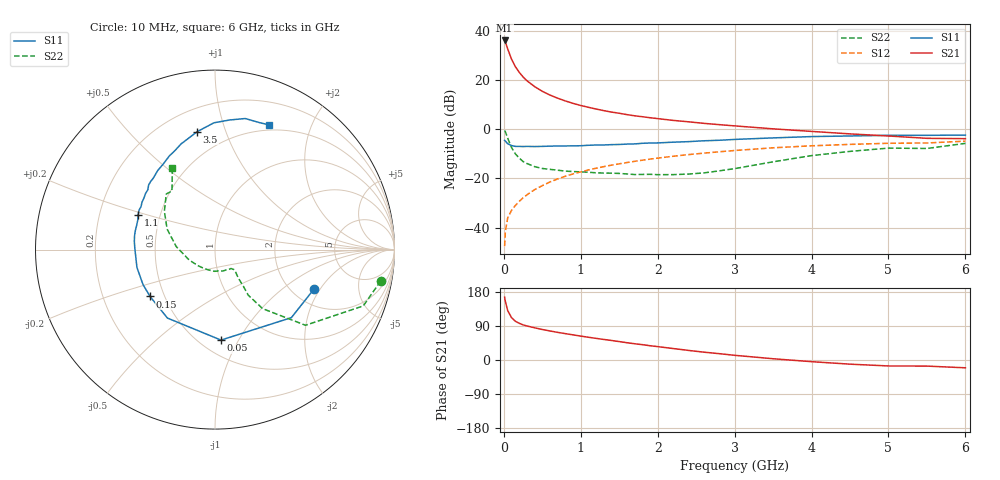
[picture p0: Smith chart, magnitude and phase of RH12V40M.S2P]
! SIEMENS Small Signal Semiconductors
! BFR106
! Si NPN RF Bipolar Junction Transistor in SOT23
! VCE = 12 V  IC = 40 mA
! Common Emitter S-Parameters:  August  1996
# GHz  S  MA  R  50
!  f  S11  S21  S12  S22
! GHz  MAG  ANG  MAG  ANG  MAG  ANG  MAG  ANG
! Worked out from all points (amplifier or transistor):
!   36 points, 10 MHz to 6 GHz, reference 50 ohm
!   highest |S21| = 36.0 dB at 10 MHz (marker M1)
!   |S21| within 3 dB of that: start of sweep to 45.39 MHz
!   unconditionally stable (mu >= 1): 304.6 MHz to 2.248 GHz
!   at 250 MHz: K = 0.96, MSG = 24.5 dB, |S12| = -27.9 dB
!   at 1.4 GHz: K = 1.07, MAG = 9.2 dB, |S12| = -14.6 dB
!   at 6 GHz: K = 0.97, MSG = 0.5 dB, |S12| = -4.9 dB
!   S11 on the Smith chart (normalised r, x): 10 MHz: 2.59, -1.76; 50 MHz: 0.63, -0.85; 150 MHz: 0.42, -0.27; 1.1 GHz: 0.37, +0.18; 3.5 GHz: 0.34, +0.80; 6 GHz: 0.44, +1.43
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0.01  0.5936 -21.8  63.31 165.8  0.0042 81.3  0.9398 -10.7
0.02  0.5698 -41.7  59.04 154.7  0.0084 71.4  0.8837 -20.8
0.05  0.5053 -86.2  42.64 130.4  0.0157 61.2  0.6571 -39.9
0.1  0.4645 -124.8  26.43 111.8  0.0224 58.0  0.4227 -51.1
0.15  0.4463 -144.2  18.54 102.2  0.0282 59.9  0.3143 -53.9
0.2  0.4459 -154.2  14.29 96.9  0.0341 62.7  0.2586 -52.3
0.25  0.4433 -162.2  11.49 92.7  0.0404 65.0  0.2197 -51.2
0.3  0.4461 -167.1  9.64 89.8  0.0463 67.0  0.2005 -50.4
0.4  0.4433 -175.2  7.316 85.0  0.059 68.8  0.1734 -47.8
0.5  0.4465 179.4  5.87 80.5  0.0712 69.4  0.159 -46.4
0.6  0.4516 174.3  4.925 76.6  0.0846 69.7  0.1526 -46.6
0.7  0.4548 170.3  4.252 72.9  0.0975 69.3  0.1466 -48.0
0.9  0.4569 162.8  3.336 66.3  0.1233 67.8  0.1376 -50.1
1.1  0.4703 155.9  2.778 60.0  0.1484 66.0  0.1331 -56.8
1.3  0.4769 149.7  2.376 54.2  0.1734 63.8  0.1285 -62.7
1.6  0.4972 141.1  1.973 45.6  0.2098 60.2  0.123 -75.4
2.2  0.5437 126.0  1.507 30.3  0.2815 52.4  0.1192 -108.3
2.8  0.5947 112.1  1.235 16.7  0.3471 44.1  0.1422 -149.8
3.5  0.6644 98.6  1.015 3.3  0.4181 34.2  0.2171 175.4
4.5  0.7269 83.5  0.802 -11.0  0.4903 19.5  0.3536 142.9
5.5  0.7498 70.5  0.651 -16.1  0.5242 9.1  0.4049 126.3
6  0.7572 66.7  0.641 -20.6  0.5701 1.9  0.5146 117.5
